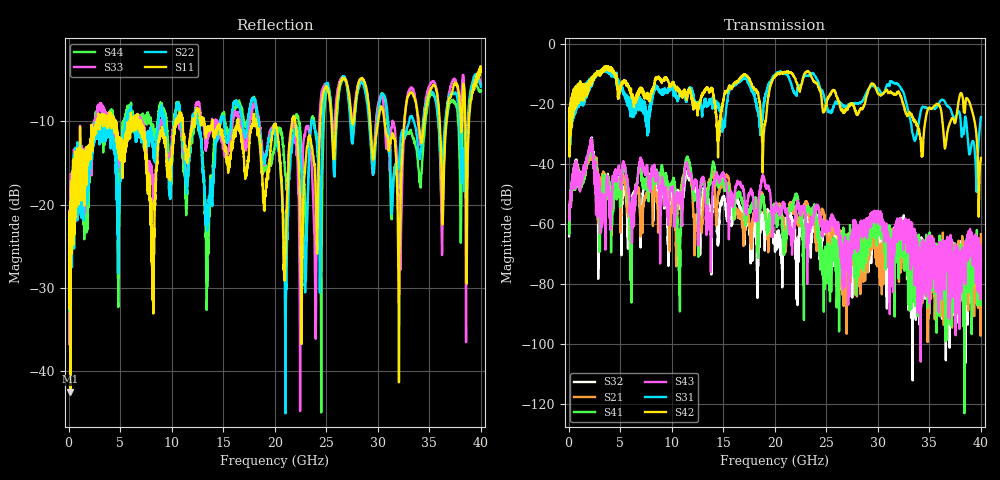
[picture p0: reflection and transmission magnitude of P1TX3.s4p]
!Agilent Technologies,N5245A,MY49151084,A.09.20.08
!Agilent N5245A: A.09.20.08
!Date: Thursday, March 01, 2012 14:25:17
!Correction: S11(Full 4 Port(1,2,3,4))
!S12(Full 4 Port(1,2,3,4))
!S13(Full 4 Port(1,2,3,4))
!S14(Full 4 Port(1,2,3,4))
!S21(Full 4 Port(1,2,3,4))
!S22(Full 4 Port(1,2,3,4))
!S23(Full 4 Port(1,2,3,4))
!S24(Full 4 Port(1,2,3,4))
!S31(Full 4 Port(1,2,3,4))
!S32(Full 4 Port(1,2,3,4))
!S33(Full 4 Port(1,2,3,4))
!S34(Full 4 Port(1,2,3,4))
!S41(Full 4 Port(1,2,3,4))
!S42(Full 4 Port(1,2,3,4))
!S43(Full 4 Port(1,2,3,4))
!S44(Full 4 Port(1,2,3,4))
!S4P File: Measurements: <S11,S12,S13,S14>,
!<S21,S22,S23,S24>,
!<S31,S32,S33,S34>,
!<S41,S42,S43,S44>:
# Hz S  dB  R 50
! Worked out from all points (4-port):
!   3996 points, 50 MHz to 40 GHz, reference 50 ohm
!   strongest paths, dB at 50 MHz, 10.04 GHz, 20.03 GHz, 30.02 GHz, 40 GHz:
!     S42: -25.4, -13.1, -10.6, -16.4, -37.9
!     S31: -25.2, -14.2, -10.3, -14.8, -24.3
!     S43: -57.2, -48.0, -55.6, -58.0, -72.4
!     S41: -60.7, -46.0, -55.9, -61.8, -73.9
!     S21: -61.8, -55.2, -54.7, -66.2, -63.3
!     S32: -64.0, -49.2, -69.2, -60.7, -71.8
!   lowest |S11| = -42.4 dB at 180 MHz (marker M1), VSWR 1.02, Z = 50.5 - j0.538 ohm
!   |S11| at or under -10 dB: start of sweep to 2.739 GHz; 6.991 GHz to 10.42 GHz (3.427 GHz wide, 39.4 % of centre); 18.14 GHz to 21.69 GHz (3.551 GHz wide, 17.8 % of centre)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
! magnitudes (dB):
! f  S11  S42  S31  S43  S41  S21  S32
! 50 MHz  -23.6  -25.4  -25.2  -57.2  -60.7  -61.8  -64.0
! 180 MHz  -42.4  -29.5  -29.4  -52.5  -51.7  -51.8  -52.5
! 2.18 GHz  -12.5  -12.7  -12.6  -31.4  -31.8  -32.2  -31.4
! 10.7 GHz  -9.2  -15.1  -17.2  -52.4  -75.4  -51.6  -50.0
! 23.19 GHz  -12.9  -8.9  -10.5  -67.3  -55.4  -53.5  -60.0
! 38.08 GHz  -11.2  -16.2  -27.9  -70.7  -71.5  -71.1  -69.5
! 40 GHz  -4.1  -37.9  -24.3  -72.4  -73.9  -63.3  -71.8
